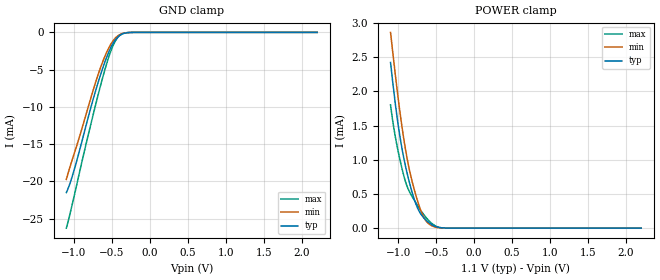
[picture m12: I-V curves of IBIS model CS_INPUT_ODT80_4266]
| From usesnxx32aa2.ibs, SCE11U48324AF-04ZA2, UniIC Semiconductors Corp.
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| CS_INPUT_ODT80_4266 (with 80ohm ODT, 3200-4266Mbps)
[Model]   CS_INPUT_ODT80_4266
Model_type   Input
Vinl = 110.833mV
Vinh = 255.833mV
|   typ   min   max
|C_comp   0.566pF   0.516pF   0.621pF
C_comp_power_clamp   0.2830pF   0.2580pF   0.3105pF
C_comp_gnd_clamp   0.2830pF   0.2580pF   0.3105pF
| Note: C_comp changes when the ODT circuit is enabled.
[Model Spec]
| Input threshold voltage corners
Vinl   0.1108V   0.1042V   0.1225V
Vinh   0.2558V   0.2492V   0.2675V
| Dynamic Overshoot Parameters from LPDDR4 Specification
D_overshoot_ampl_h   0.30   NA   NA
D_overshoot_ampl_l   0.30   NA   NA
D_overshoot_area_h   0.1n   NA   NA
D_overshoot_area_l   0.1n   NA   NA
[Receiver Thresholds]
Vth   = 0.1833V
Vth_min  = 0.1800V
Vth_max  = 0.1866V
Vinh_ac  = 0.072V
Vinh_dc  = 0.072V
Vinl_ac  = -0.072V
Vinl_dc  = -0.072V
Tslew_ac = 5.000ns |Not specified, so set to high value
Threshold_sensitivity = 0.1667
Reference_supply Power_clamp_ref
[Voltage Range]   1.1000V   1.0600V   1.1700V
[POWER Clamp Reference]   1.1000V   1.0600V   1.1700V
| Junction Temperature (Ambient temp is 35C typ 95C min -40C max)
[Temperature Range]   50.0   110.0   -40.0
[Add Submodel]
| Submodel Name   Mode
80ohm_ODT_4266   Non-Driving
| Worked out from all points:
|   GND clamp passes 1 mA (typ) near -0.45 V on its own axis
|   POWER clamp passes 1 mA (typ) near -0.92 V on its own axis
[GND Clamp]
|   Voltage   I(typ)   I(min)   I(max)
-1.1V     -21.5mA    -19.74mA   -26.28mA
-1.05V    -20.21mA   -18mA      -24.3mA
-1.001V   -18.6mA    -16.41mA   -22.15mA
-756.8mV  -9.324mA   -8.096mA   -11.46mA
-674.3mV  -6.48mA    -5.435mA   -8.091mA
-611.6mV  -4.527mA   -3.692mA   -5.689mA
-545.6mV  -2.746mA   -2.177mA   -3.434mA
-486.2mV  -1.497mA   -1.155mA   -1.803mA
-436.7mV  -775.7uA   -585.7uA   -864uA
-387.2mV  -339.6uA   -253.2uA   -334.1uA
-199.1mV  -2.761uA   -2.971uA   -1.176uA
2.2V      0A         0A         0A
[POWER Clamp]
|   Voltage   I(typ)   I(min)   I(max)
-1.1V     2.422mA    2.862mA    1.802mA
-1.041V   1.852mA    2.278mA    1.359mA
-981.2mV  1.374mA    1.741mA    1.027mA
-921.8mV  1.005mA    1.277mA    751.6uA
-862.4mV  713uA      909uA      558.8uA
-783.2mV  406.4uA    545.8uA    401.7uA
-710.6mV  222.9uA    283.8uA    272.7uA
-657.8mV  145uA      149.1uA    190.2uA
-591.8mV  77.53uA    58.55uA    105.1uA
-486.2mV  16.52uA    9.628uA    20.62uA
-370.7mV  1.13uA     773.1nA    818.4nA
2.2V      0A         0A         0A
